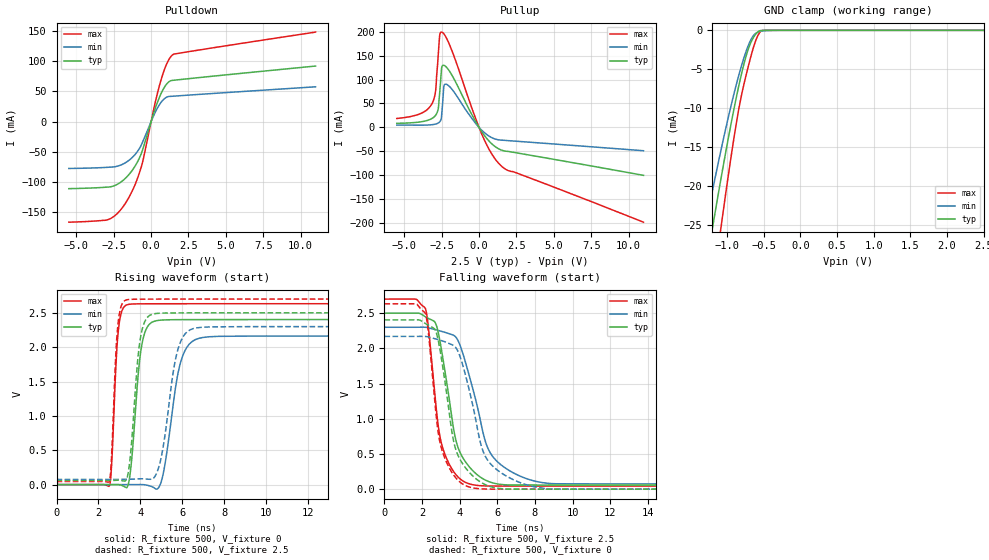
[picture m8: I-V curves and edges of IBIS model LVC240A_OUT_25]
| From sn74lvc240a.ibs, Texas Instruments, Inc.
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[Model]   LVC240A_OUT_25
Model_type  3-state
Enable   Active-Low
Vref =   0
Rref =   500
Cref =   30p
Vmeas =   1.25
| variable   typ   min   max
C_comp   5.31pF   5.03pF   5.82pF
| C_pullup   7.01pF   5.85pF   7.58pF
| C_pulldown   6.47pF   5.12pF   7.86pF
| C_tri-state   5.31pF   5.03pF   5.82pF
[Temperature Range]   40   100   -40
| Ambient temperature   25   85   -40
[Voltage range]   2.5   2.3   2.7
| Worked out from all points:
|   slope of the pulldown table from 0 to 0.375 V, typ, clamps not added: 13 ohm
|   slope of the pullup table from 0 to 0.375 V, typ, clamps not added: 21.5 ohm
|   GND clamp passes 1 mA (typ) near -0.64 V on its own axis
|   rising waveform, R_fixture 500, V_fixture 0: 20-80 % time 392ps typ, 632ps min, 241ps max; typ from 0 V to 2.4 V
|   falling waveform, R_fixture 500, V_fixture 2.5: 20-80 % time 967ps typ, 1.37ns min, 723ps max; typ from 2.5 V to 0.058 V
|   rising waveform, R_fixture 500, V_fixture 2.5: 20-80 % time 384ps typ, 628ps min, 233ps max; typ from 0.058 V to 2.5 V
|   falling waveform, R_fixture 500, V_fixture 0: 20-80 % time 921ps typ, 1.24ns min, 712ps max; typ from 2.4 V to 0 V
[GND Clamp]
| LVC240A_OUT_25
|   Voltage   I(typ)   I(min)   I(max)
-5.5V     -311.6mA   -259.3mA   -396.4mA
-1.31V    -31.75mA   -25.83mA   -41.58mA
-1.265V   -29.16mA   -23.69mA   -38.28mA
-1.22V    -26.61mA   -21.59mA   -35.01mA
-1.175V   -24.09mA   -19.52mA   -31.79mA
-1.095V   -19.72mA   -15.94mA   -26.19mA
-1.06V    -17.86mA   -14.42mA   -23.79mA
-875mV    -8.7mA     -7.025mA   -12.04mA
-760mV    -3.983mA   -3.255mA   -6.545mA
-650mV    -1.084mA   -807.5uA   -2.519mA
-535mV    -25.82uA   -102.9uA   -89.75uA
2.5V      48.15pA    25.99nA    -1.562nA
[Pulldown]
| LVC240A_OUT_25
|   Voltage   I(typ)   I(min)   I(max)
-5.5V     -110.9mA   -77.52mA   -166.4mA
-2.86V    -108.3mA   -75.52mA   -162mA
-2.255V   -103.7mA   -73.72mA   -151.9mA
-1.655V   -92.21mA   -67.04mA   -132.6mA
-1.13V    -75.85mA   -56.02mA   -107.5mA
-700mV    -55.51mA   -40.79mA   -78.33mA
-525mV    -43.32mA   -31.25mA   -62.33mA
245mV     19.49mA    13.85mA    28.34mA
595mV     42.54mA    29.39mA    62.99mA
1.03V     61.88mA    40.37mA    94.77mA
1.435V    68.29mA    42.04mA    110.4mA
11V       91.99mA    57.63mA    148.2mA
[Pullup]
| LVC240A_OUT_25
|   Voltage   I(typ)   I(min)   I(max)
-5.5V     8.51mA     4.863mA    18.58mA
-3.91V    11.55mA    4.714mA    28.82mA
-3.14V    18.79mA    5.666mA    49.97mA
-2.905V   25.32mA    6.979mA    75.87mA
-2.73V    38.61mA    9.098mA    150.1mA
-2.625V   74.51mA    11.69mA    193.3mA
-2.475V   127.2mA    34.48mA    198.8mA
-2.35V    129.6mA    86.31mA    195.3mA
-2.145V   124.6mA    89.55mA    184.5mA
185mV     -9.092mA   -6.052mA   -14.17mA
1.465V    -46.97mA   -26.57mA   -79.91mA
11V       -100.1mA   -48.72mA   -197.9mA
[Ramp]
| LVC240A_OUT_25
| variable   typ   min   max
dV/dt_r   1.47/4.08E-10   1.34/6.51E-10   1.59/2.52E-10
dV/dt_f   1.47/9.72E-10   1.34/1.37E-09   1.59/7.27E-10
R_load = 500
[Rising Waveform]
| LVC240A_OUT_25
R_fixture =   500
C_fixture =   0
L_fixture =   0
V_fixture =   0
V_fixture_min = 0
V_fixture_max = 0
|   Time   V(typ)   V(min)   V(max)
0s        750.8pV    3.045nV    27.79nV
2.53ns    -447.2uV   -182.4uV   -13.23mV
2.94ns    -703.8uV   -380.8uV   2.218V
3.425ns   8.897mV    -284.4uV   2.622V
4.07ns    2.038V     -220.6uV   2.631V
4.8ns     2.387V     -63.9mV    2.632V
5.125ns   2.396V     216.8mV    2.632V
5.935ns   2.4V       1.8V       2.632V
6.985ns   2.401V     2.141V     2.632V
50ns      2.402V     2.163V     2.632V
[Falling Waveform]
| LVC240A_OUT_25
R_fixture =   500
C_fixture =   0
L_fixture =   0
V_fixture =   2.5
V_fixture_min = 2.3
V_fixture_max = 2.7
|   Time   V(typ)   V(min)   V(max)
0s        2.5V       2.3V       2.7V
2.18ns    2.449V     2.3V       2.563V
2.7ns     2.365V     2.267V     1.3V
3.065ns   1.927V     2.239V     616.4mV
3.805ns   689.2mV    2.157V     204.9mV
4.7ns     261.6mV    1.425V     63.01mV
5.345ns   132.1mV    697.7mV    46.43mV
5.78ns    87.71mV    456mV      44.64mV
8.615ns   58.55mV    85.65mV    44.09mV
50ns      58.46mV    74.55mV    43.93mV
[Rising Waveform]
| LVC240A_OUT_25
R_fixture =   500
C_fixture =   0
L_fixture =   0
V_fixture =   2.5
V_fixture_min = 2.3
V_fixture_max = 2.7
|   Time   V(typ)   V(min)   V(max)
0s        58.44mV    74.47mV    43.92mV
2.52ns    59.11mV    74.31mV    46.72mV
2.925ns   63.31mV    74.85mV    2.319V
3.375ns   107.3mV    76.45mV    2.691V
4ns       2.131V     84.49mV    2.699V
4.685ns   2.487V     115mV      2.699V
5.05ns    2.496V     487.3mV    2.7V
5.785ns   2.498V     1.964V     2.7V
6.695ns   2.499V     2.282V     2.7V
50ns      2.5V       2.3V       2.7V
[Falling Waveform]
| LVC240A_OUT_25
R_fixture =   500
C_fixture =   0
L_fixture =   0
V_fixture =   0
V_fixture_min = 0
V_fixture_max = 0
|   Time   V(typ)   V(min)   V(max)
0s        2.405V     2.17V      2.633V
2.18ns    2.352V     2.17V      2.492V
2.685ns   2.266V     2.138V     1.229V
3.01ns    1.891V     2.112V     600.9mV
3.725ns   628.6mV    2.031V     183.8mV
4.69ns    189.6mV    1.199V     19.11mV
5.16ns    92.93mV    606.7mV    4.547mV
5.615ns   38.13mV    367.4mV    1.009mV
8.54ns    113.2uV    9.385mV    169uV
50ns      24.41uV    73.09uV    7.871uV
